(* Logix 5000 AddOnInstructionDefinition export AMCI_3202_AOP_Hold; software revision 20.03 *)

ADD_ON_INSTRUCTION AMCI_3202_AOP_Hold   (* revision 1.0, vendor AMCI, ExecuteEnableInFalse *)
VAR_INPUT
   channel_number : INT; {required}
END_VAR
VAR_IN_OUT
   AMCI_3202_output_data : AM:1756_3202:O:0; {required}
END_VAR
VAR
   command_data_block : DINT[8]; {access None}
END_VAR

ROUTINE EnableInFalse   (* ladder *)
END_ROUTINE

ROUTINE Logic   (* ladder *)
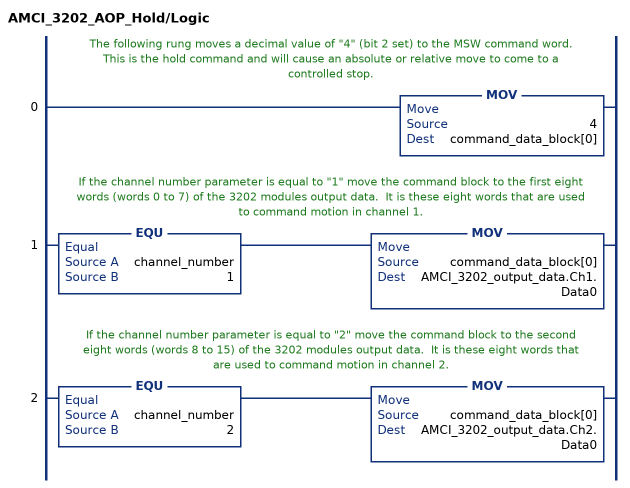
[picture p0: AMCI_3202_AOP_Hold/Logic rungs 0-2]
   // The following rung moves a decimal value of "4" (bit 2 set) to the MSW command word.  This is the hold command and will cause an absolute or relative move to come to a controlled stop.
   0: MOV(4,command_data_block[0]);
   // If the channel number parameter is equal to "1" move the command block to the first eight words (words 0 to 7) of the 3202 modules output data.  It is these eight words that are used to command motion in channel 1.
   1: EQU(channel_number,1)MOV(command_data_block[0],AMCI_3202_output_data.Ch1.Data0);
   // If the channel number parameter is equal to "2" move the command block to the second eight words (words 8 to 15) of the 3202 modules output data.  It is these eight words that are used to command motion in channel 2.
   2: EQU(channel_number,2)MOV(command_data_block[0],AMCI_3202_output_data.Ch2.Data0);
END_ROUTINE
END_ADD_ON_INSTRUCTION
